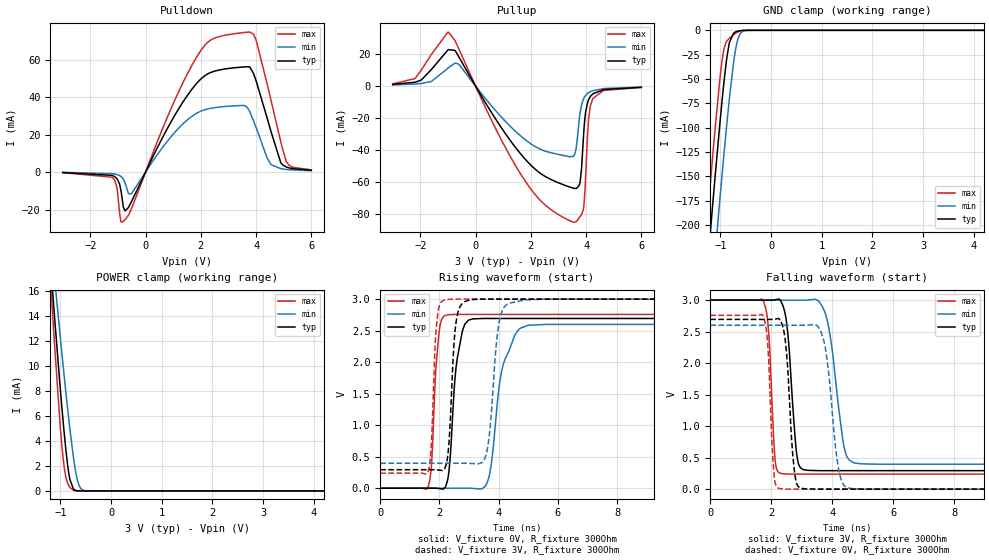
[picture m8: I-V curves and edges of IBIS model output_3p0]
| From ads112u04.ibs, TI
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|   output_3p0 Model
[Model]   output_3p0
Model_type   3-state
Polarity   Non-Inverting
Vmeas = 1.5
Vref = 0
Cref = 2pF
Rref = 100000
|   typ   min   max
C_comp   1.43758E-12   1.43753E-12   1.45091E-12
|C_comp_pullup   1.22358E-12   1.22356E-12   1.22925E-12
|C_comp_pulldown   1.14724E-12   1.13137E-12   1.2124E-12
| Where Nom  PVT is Nominal Process, 3.0V, 27C
|   Fast PVT is Strong Process,  3.001V, -40C
|   Slow PVT is Weak Process,   2.999, 125C
[Voltage Range]   3   2.999   3.001
[Temperature Range]   27   125   -40
[Pullup Reference]   3   2.999   3.001
[Pulldown Reference]   0   0   0
[Power Clamp Reference]   3   2.999   3.001
[GND Clamp Reference]   0   0   0
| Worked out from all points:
|   slope of the pulldown table from 0 to 0.45 V, typ, clamps not added: 32.9 ohm
|   slope of the pullup table from 0 to 0.45 V, typ, clamps not added: 34.5 ohm
|   GND clamp passes 1 mA (typ) near -0.67 V on its own axis
|   POWER clamp passes 1 mA (typ) near -0.82 V on its own axis
|   falling waveform, V_fixture 3V, R_fixture 300Ohm: 20-80 % time 235ps typ, 394ps min, 162ps max; typ from 3 V to 0.293 V
|   rising waveform, V_fixture 0V, R_fixture 300Ohm: 20-80 % time 268ps typ, 460ps min, 181ps max; typ from 0 V to 2.69 V
|   rising waveform, V_fixture 3V, R_fixture 300Ohm: 20-80 % time 182ps typ, 265ps min, 141ps max; typ from 0.293 V to 3 V
|   falling waveform, V_fixture 0V, R_fixture 300Ohm: 20-80 % time 205ps typ, 324ps min, 150ps max; typ from 2.69 V to 0 V
[Pulldown]
|   Voltage   I(typ)   I(min)   I(max)
-3V       -273.9uA   -170.1uA   -318.1uA
-1.209V   -1.837mA   -882.3uA   -2.871mA
-1.038V   -3.53mA    -1.358mA   -8.223mA
-948mV    -6.152mA   -1.85mA    -20.51mA
-804mV    -18.75mA   -3.787mA   -26.32mA
-525mV    -16.24mA   -11.64mA   -20.1mA
1.977V    49.29mA    32.32mA    64.32mA
3.75V     56.09mA    32.76mA    74.65mA
3.993V    48.97mA    24.06mA    70.62mA
4.542V    21.51mA    3.966mA    38.21mA
5.091V    2.699mA    1.387mA    5.654mA
6V        980.2uA    687.2uA    1.154mA
[GND Clamp]
|   Voltage   I(typ)   I(min)   I(max)
-3V       -1.375A    -1.451A    -1.328A
-1.317V   -280.6mA   -360.8mA   -230.1mA
-1.164V   -185.9mA   -265.9mA   -135.8mA
-1.11V    -153.4mA   -233mA     -103.9mA
-1.011V   -96.01mA   -173.8mA   -50.17mA
-930mV    -53.23mA   -127.2mA   -19.2mA
-876mV    -29.27mA   -97.52mA   -11.32mA
-822mV    -12.5mA    -69.61mA   -8.069mA
-696mV    -1.513mA   -18.47mA   -2.875mA
-615mV    -369.7uA   -4.096mA   -852.1uA
-480mV    -14.73uA   -138.7uA   -25.12uA
6V        0A         0A         0A
[Pullup]
|   Voltage   I(typ)   I(min)   I(max)
-3V       1.091mA    745.1uA    1.366mA
-2.19V    2.436mA    1.303mA    4.756mA
-984mV    22.89mA    11.5mA     33.86mA
-615mV    18.63mA    13.82mA    23.65mA
1.779V    -45.45mA   -33.32mA   -59.05mA
3.561V    -64.06mA   -43.67mA   -85.27mA
3.786V    -59.69mA   -16.41mA   -81.68mA
3.903V    -32.61mA   -8.185mA   -77.23mA
3.984V    -16.32mA   -5.811mA   -57.08mA
4.092V    -8.528mA   -4.11mA    -20.62mA
4.245V    -4.854mA   -2.861mA   -7.751mA
6V        -745.7uA   -590.3uA   -837.5uA
[POWER Clamp]
|   Voltage   I(typ)   I(min)   I(max)
-3V       122.5mA    105.5mA    143.2mA
-1.182V   17.52mA    19.99mA    16.03mA
-1.164V   16.54mA    19.2mA     14.87mA
-1.128V   14.62mA    17.64mA    12.56mA
-1.11V    13.67mA    16.87mA    11.43mA
-1.002V   8.181mA    12.32mA    5.126mA
-930mV    4.862mA    9.397mA    2.035mA
-840mV    1.556mA    5.942mA    465.8uA
-741mV    140.2uA    2.648mA    45.44uA
-633mV    6.42uA     466.3uA    1.703uA
-498mV    124.3nA    13.54uA    0A
6V        0A         0A         0A
[Ramp]
R_load = 300
|   typ   min   max
dV/dt_r   1.6162/2.67708e-10   1.56008/4.59201e-10   1.65491/1.80957e-10
dV/dt_f   1.62405/2.35386e-10   1.56183/3.93376e-10   1.65761/1.61671e-10
[Falling Waveform]
V_fixture = 3V
V_fixture_min = 2.999V
V_fixture_max = 3.001V
R_fixture = 300Ohm
C_fixture = 0F
|   Time   V(typ)   V(min)   V(max)
0s        3V         2.999V     3.001V
1.748ns   2.999V     2.998V     2.976V
2.13ns    3.005V     2.998V     439.3mV
2.374ns   2.916V     2.998V     243.6mV
2.84ns    520.5mV    2.998V     238.7mV
3.197ns   298.4mV    3.001V     238.7mV
3.768ns   293.7mV    2.788V     238.6mV
4.397ns   293.7mV    637.6mV    238.6mV
4.934ns   293.7mV    402.6mV    238.6mV
50ns      293.2mV    396mV      238.3mV
[Rising Waveform]
V_fixture = 0V
V_fixture_min = 0V
V_fixture_max = 0V
R_fixture = 300Ohm
C_fixture = 0F
|   Time   V(typ)   V(min)   V(max)
0s        -50.7nV    -132.2nV   -25.55nV
1.613ns   743.6uV    416.7uV    16.69mV
1.975ns   -4.755mV   510.3uV    2.421V
2.273ns   126.8mV    587.2uV    2.752V
2.608ns   2.079V     673.9uV    2.758V
3.132ns   2.687V     -3.457mV   2.758V
3.644ns   2.693V     131.7mV    2.758V
4.125ns   2.693V     1.91V      2.758V
4.993ns   2.693V     2.585V     2.758V
50ns      2.694V     2.6V       2.758V
[Rising Waveform]
V_fixture = 3V
V_fixture_min = 2.999V
V_fixture_max = 3.001V
R_fixture = 300Ohm
C_fixture = 0F
|   Time   V(typ)   V(min)   V(max)
0s        293.2mV    396mV      238.3mV
1.604ns   293.8mV    396.1mV    251mV
1.918ns   291.5mV    396.1mV    2.664V
2.219ns   361.5mV    396.1mV    2.994V
2.563ns   2.642V     396.1mV    3.001V
3.048ns   2.992V     393.4mV    3.001V
3.6ns     3V         576.6mV    3.001V
4.104ns   3V         2.796V     3.001V
4.881ns   3V         2.988V     3.001V
50ns      3V         2.999V     3.001V
[Falling Waveform]
|Gnd
V_fixture = 0V
V_fixture_min = 0V
V_fixture_max = 0V
R_fixture = 300Ohm
C_fixture = 0F
|   Time   V(typ)   V(min)   V(max)
0s        2.694V     2.6V       2.758V
1.73ns    2.693V     2.6V       2.749V
2.092ns   2.696V     2.6V       215.5mV
2.351ns   2.616V     2.6V       4.267mV
2.774ns   220.8mV    2.6V       386.4uV
3.103ns   4.731mV    2.6V       386.2uV
3.692ns   412.2uV    2.406V     386uV
4.228ns   412uV      261.6mV    385.8uV
4.698ns   411.8uV    6.11mV     385.6uV
50ns      -51.4nV    -132.8nV   -26.14nV
